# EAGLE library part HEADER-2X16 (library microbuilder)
PIN HEADER
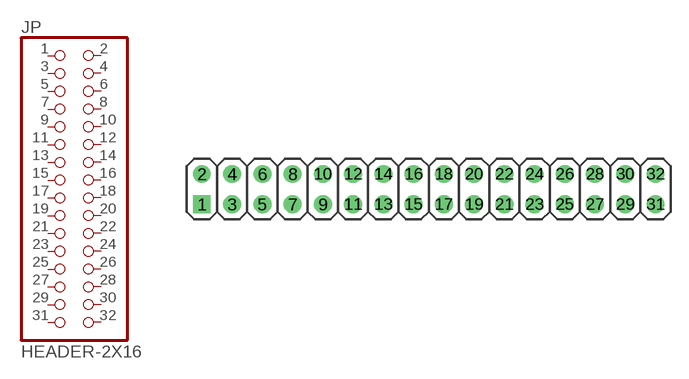
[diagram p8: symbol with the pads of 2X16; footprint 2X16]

Designator prefix JP

## HEADER-2X16  [2X16]
1  1  pas
2  2  pas
3  3  pas
4  4  pas
5  5  pas
6  6  pas
7  7  pas
8  8  pas
9  9  pas
10  10  pas
11  11  pas
12  12  pas
13  13  pas
14  14  pas
15  15  pas
16  16  pas
17  17  pas
18  18  pas
19  19  pas
20  20  pas
21  21  pas
22  22  pas
23  23  pas
24  24  pas
25  25  pas
26  26  pas
27  27  pas
28  28  pas
29  29  pas
30  30  pas
31  31  pas
32  32  pas

## Footprint 2X16 (pad centres in mm)
PIN HEADER
drill 1 square: 1 -19.05,-1.27
drill 1: 2 -19.05,1.27; 3 -16.51,-1.27; 4 -16.51,1.27; 5 -13.97,-1.27; 6 -13.97,1.27; 7 -11.43,-1.27; 8 -11.43,1.27; 9 -8.89,-1.27; 10 -8.89,1.27; 11 -6.35,-1.27; 12 -6.35,1.27; 13 -3.81,-1.27; 14 -3.81,1.27; 15 -1.27,-1.27; 16 -1.27,1.27; 17 1.27,-1.27; 18 1.27,1.27; 19 3.81,-1.27; 20 3.81,1.27; 21 6.35,-1.27; 22 6.35,1.27; 23 8.89,-1.27; 24 8.89,1.27; 25 11.43,-1.27; 26 11.43,1.27; 27 13.97,-1.27; 28 13.97,1.27; 29 16.51,-1.27; 30 16.51,1.27; 31 19.05,-1.27; 32 19.05,1.27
